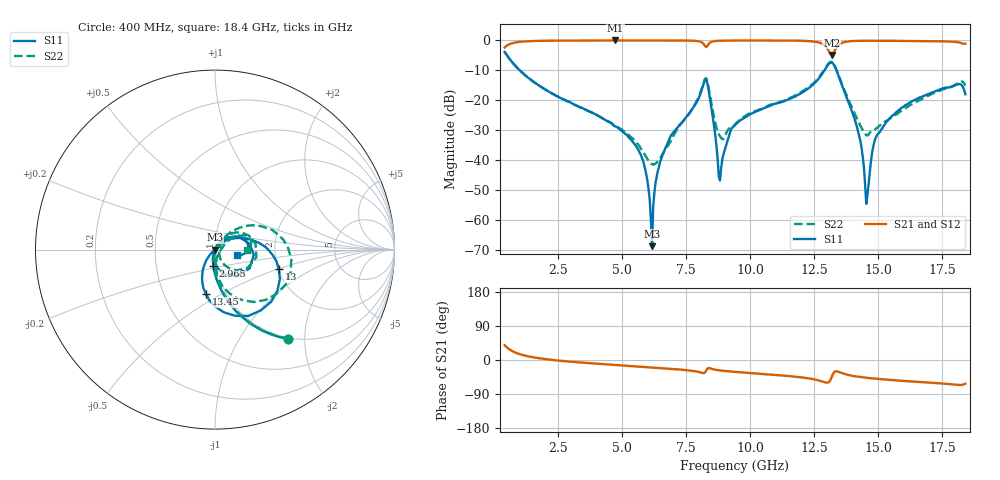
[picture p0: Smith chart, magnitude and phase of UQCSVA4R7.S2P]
!  Part Number  UQCSVA4R7  Mounting Orientation: Horizontal
!  Description: Ultra Low ESR Microwave capacitors
!  Application: Coupling, Bypass, Tuning, DC Block
!  Filters, Matching
# GHZ S DB R 50
! Freq  |S11|  S11 Ph  |S21|  S21 Ph  |S12|  S12 Ph  |S22|  S22 Ph
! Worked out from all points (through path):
!   401 points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, 400 MHz to 18.4 GHz, reference 50 ohm
!   highest |S21| = -0.01 dB at 4.72 GHz (marker M1); lowest = -4.8 dB at 13.18 GHz (marker M2)
!   group delay of S21, straight-line fit = 11.7 ps
!   lowest |S11| = -68.8 dB at 6.16 GHz (marker M3), VSWR 1.00, Z = 50 + j0.0253 ohm
!   |S11| at or under -10 dB: 992.9 MHz to 12.89 GHz (11.9 GHz wide, 171 % of centre); 13.36 GHz to end of sweep
!   |S22| runs from -41.5 to -3.8 dB; largest |S21 - S12| = 0.0077
!   S11 on the Smith chart (normalised r, x): 400 MHz: 0.98, -1.66; 2.965 GHz: 0.96, -0.18; 13 GHz: 2.02, -0.51; 13.45 GHz: 0.80, -0.42; 18.4 GHz: 1.28, -0.07
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0.4  -3.84 -50.5  -2.39 38.9  -2.39 38.8  -3.84 -50.6
1.12  -11.03 -77.0  -0.38 12.9  -0.38 12.7  -11.01 -76.7
2.965  -20.69 -96.0  -0.05 -4.5  -0.05 -4.5  -20.74 -92.2
3.415  -22.54 -98.6  -0.04 -6.9  -0.05 -7.0  -22.58 -92.7
4.72  -28.71 -104.6  -0.01 -13.3  -0.02 -13.4  -28.38 -93.9
5.71  -38.03 -111.8  -0.01 -17.9  -0.02 -18.0  -35.95 -82.1
6.16  -68.75 43.7  -0.02 -20.0  -0.02 -20.1  -41.32 -34.5
6.43  -42.30 64.5  -0.02 -21.3  -0.03 -21.3  -39.95 9.2
8.23  -13.22 -7.7  -1.88 -33.0  -1.87 -32.9  -12.82 7.8
8.41  -18.76 -78.5  -0.82 -21.6  -0.83 -21.6  -17.77 -53.1
8.815  -46.80 -3.4  -0.11 -27.7  -0.11 -27.7  -32.02 -20.2
9.4  -28.29 53.7  -0.06 -31.4  -0.07 -31.4  -28.08 42.6
12.415  -15.03 20.6  -0.33 -50.0  -0.32 -50.0  -14.64 41.4
13  -8.59 -17.2  -2.63 -59.7  -2.62 -59.7  -8.28 8.1
13.18  -7.45 -53.0  -4.82 -44.6  -4.81 -44.8  -7.14 -26.3
13.45  -11.98 -101.8  -1.55 -31.2  -1.54 -31.2  -11.73 -71.3
14.215  -30.62 -135.9  -0.14 -44.2  -0.14 -44.2  -27.10 -75.6
14.53  -54.62 -63.8  -0.10 -47.0  -0.10 -47.0  -31.68 -39.0
14.89  -32.65 41.3  -0.09 -49.2  -0.11 -49.2  -29.62 -1.3
15.43  -26.21 40.8  -0.11 -52.3  -0.12 -52.3  -26.22 20.4
17.455  -16.23 26.2  -0.30 -62.0  -0.28 -61.6  -16.59 31.1
18.4  -18.01 -12.7  -1.08 -62.6  -1.02 -62.5  -15.07 -0.1
